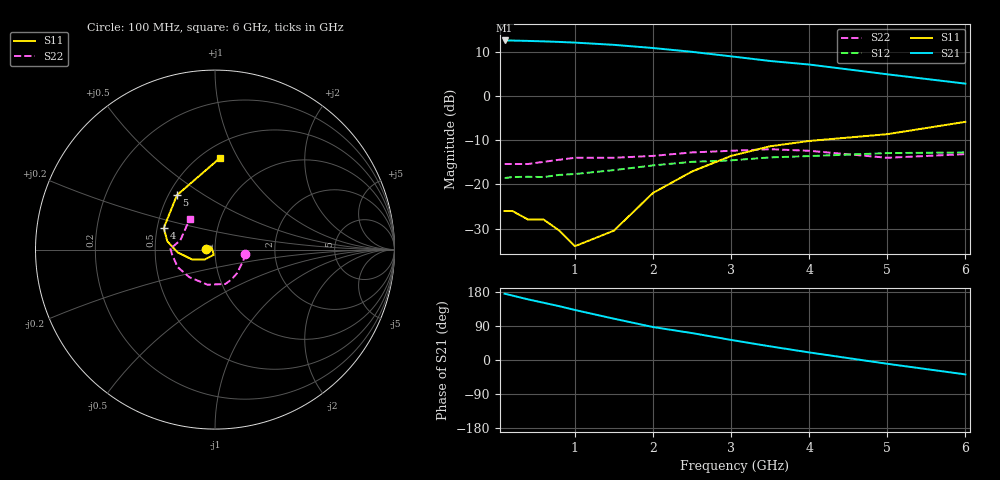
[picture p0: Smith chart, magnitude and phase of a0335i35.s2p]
!  MSA-0335 S AND NOISE PARAMETERS
!  Id=35mA  LAST UPDATED 07-22-92
# ghz s ma r 50
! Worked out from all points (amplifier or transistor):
!   14 points, 100 MHz to 6 GHz, reference 50 ohm
!   highest |S21| = 12.6 dB at 100 MHz (marker M1)
!   |S21| within 3 dB of that: start of sweep to 2.709 GHz
!   unconditionally stable (mu >= 1): start of sweep to end of sweep
!   at 400 MHz: K = 1.20, MAG = 12.7 dB, |S12| = -18.3 dB
!   at 2 GHz: K = 1.10, MAG = 11.4 dB, |S12| = -15.7 dB
!   at 6 GHz: K = 1.25, MAG = 4.8 dB, |S12| = -12.8 dB
!   lowest NFmin = 5.60 dB at 100 MHz
!   S11 on the Smith chart (normalised r, x): 100 MHz: 0.90, +0.00; 4 GHz: 0.54, +0.15; 5 GHz: 0.55, +0.39; 6 GHz: 0.61, +0.84
0.1  0.05 177.0  4.25 175.0  0.118 1.0  0.17 -8.0
0.2  0.05 170.0  4.24 170.0  0.121 2.0  0.17 -17.0
0.4  0.04 161.0  4.2 160.0  0.122 3.0  0.17 -33.0
0.6  0.04 156.0  4.15 151.0  0.121 5.0  0.18 -47.0
0.8  0.03 149.0  4.09 142.0  0.128 8.0  0.19 -61.0
1  0.02 154.0  4.02 132.0  0.131 9.0  0.2 -73.0
1.5  0.03 -104.0  3.79 109.0  0.145 13.0  0.2 -102.0
2  0.08 -136.0  3.49 87.0  0.164 11.0  0.21 -133.0
2.5  0.14 -157.0  3.16 71.0  0.18 13.0  0.23 -155.0
3  0.21 -176.0  2.81 53.0  0.187 8.0  0.24 -173.0
3.5  0.27 170.0  2.49 36.0  0.202 4.0  0.25 178.0
4  0.31 157.0  2.27 20.0  0.209 -1.0  0.24 177.0
5  0.37 125.0  1.76 -10.0  0.226 -12.0  0.2 165.0
6  0.51 87.0  1.38 -38.0  0.23 -25.0  0.22 130.0
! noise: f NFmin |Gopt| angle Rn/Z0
0.1  5.6  0.05  -1  0.84
0.5  5.8  0.05  -1  0.84
1  6  0.04  -21  0.83
2  6.5  0.04  -92  0.81
